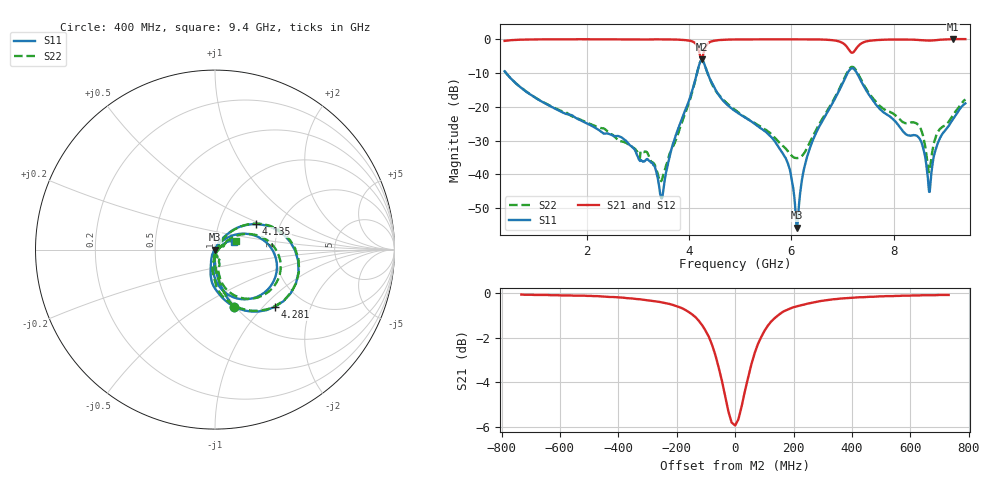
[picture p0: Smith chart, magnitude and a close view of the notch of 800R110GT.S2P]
!  American Technical Ceramics  Date:  10/25/10
!  One Norden Lane
!  Huntington Station,  NY.  11746-2102
!  Tel:  (631) 622-4700  Fax:  (631) 622-4748
!  Part Number  800R110GT.TXT  Mounting Orientation: Horizontal
!  Description: Ultra Low ESR Microwave Capacitor
!  Application: Coupling, Bypass, Tuning, DC Block, Filters, Matching
# GHZ S DB R 50
! Freq  |S11|  S11 Ph  |S21|  S21 Ph  |S12|  S12 Ph  |S22|  S22 Ph
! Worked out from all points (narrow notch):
!   801 points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, 400 MHz to 9.4 GHz, reference 50 ohm
!   highest |S21| = 0.00 dB at 9.164 GHz (marker M1); lowest = -5.9 dB at 4.248 GHz (marker M2)
!   notch at M2: 5.8 dB deep, 122 MHz wide at half that depth
!   lowest |S11| = -55.7 dB at 6.104 GHz (marker M3), VSWR 1.00, Z = 49.8 + j0.0436 ohm
!   |S11| at or under -10 dB: 426.1 MHz to 4.158 GHz (3.732 GHz wide, 163 % of centre); 4.363 GHz to 7.1 GHz (2.737 GHz wide, 47.8 % of centre); 7.279 GHz to end of sweep
!   |S22| runs from -42.2 to -6.2 dB; largest |S21 - S12| = 0.0019
!   S11 on the Smith chart (normalised r, x): 400 MHz: 0.98, -0.70; 4.135 GHz: 1.51, +0.46; 4.281 GHz: 1.44, -1.17; 9.4 GHz: 1.23, +0.10
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0.4  -9.51 -71.9  -0.53 17.8  -0.53 17.8  -9.47 -71.9
1.908  -24.17 -93.4  -0.05 -4.8  -0.04 -4.8  -23.98 -93.2
2.729  -29.56 -90.7  -0.08 -10.2  -0.07 -10.2  -30.41 -90.8
3.404  -42.10 -58.1  -0.06 -14.8  -0.06 -14.8  -40.51 -49.0
3.483  -46.52 12.8  -0.07 -15.7  -0.07 -15.7  -41.05 2.0
4.135  -11.36 31.7  -1.45 -32.2  -1.44 -32.2  -11.57 33.4
4.248  -6.22 -22.5  -5.93 -15.4  -5.93 -15.5  -6.21 -21.2
4.281  -6.71 -43.6  -4.42 -0.3  -4.42 -0.4  -6.70 -42.5
4.45  -12.98 -88.7  -0.64 -6.7  -0.64 -6.8  -13.27 -86.7
4.9  -21.26 -105.6  -0.11 -15.8  -0.11 -15.8  -20.94 -98.8
5.868  -34.64 -121.1  -0.08 -23.2  -0.07 -23.3  -32.05 -75.2
6.104  -55.71 164.5  -0.06 -25.0  -0.06 -25.1  -35.18 -33.3
6.408  -30.35 59.0  -0.07 -27.8  -0.07 -27.8  -29.13 27.6
6.993  -13.38 23.4  -1.07 -38.9  -1.07 -38.9  -13.00 22.5
7.173  -8.65 -24.4  -3.98 -31.4  -3.99 -31.5  -8.25 -21.1
7.409  -13.73 -83.5  -0.96 -17.9  -0.97 -18.0  -13.30 -75.6
7.904  -22.61 -90.9  -0.14 -26.9  -0.15 -26.9  -21.36 -72.3
8.5  -29.32 -77.0  -0.26 -32.2  -0.26 -32.2  -25.75 -67.5
8.691  -45.11 -40.7  -0.44 -31.9  -0.45 -31.9  -39.35 -24.0
8.871  -30.39 30.5  -0.25 -31.3  -0.26 -31.3  -27.22 22.4
9.164  -23.48 33.2  0.00 -32.7  -0.01 -32.8  -22.26 32.0
9.4  -18.99 21.7  -0.01 -34.7  -0.01 -34.7  -17.83 22.6
